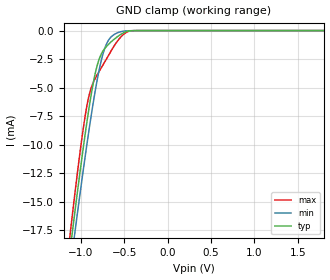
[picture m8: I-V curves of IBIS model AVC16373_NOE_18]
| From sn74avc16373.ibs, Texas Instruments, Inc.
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[Model]   AVC16373_NOE_18
Model_type  Input
Vinl=0.5775
Vinh=1.2675
| variable   typ   min   max
C_comp   1.78pF   1.31pF   2.34pF
[Temperature Range]   40   100   -40
| Ambient temperature   25   85   -40
[Voltage range]   1.8   1.65   1.95
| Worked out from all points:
|   GND clamp passes 1 mA (typ) near -0.65 V on its own axis
[GND Clamp]
| AVC16373_NOE_18
|   Voltage   I(typ)   I(min)   I(max)
-1.8V     -63.88mA   -63.41mA   -65.81mA
-1.125V   -19.32mA   -20.97mA   -17.91mA
-1.095V   -17.47mA   -19.2mA    -15.95mA
-1.065V   -15.65mA   -17.45mA   -14.03mA
-935mV    -8.251mA   -10.21mA   -6.785mA
-890mV    -6.02mA    -7.895mA   -5.239mA
-830mV    -3.604mA   -5.085mA   -4.126mA
-780mV    -2.319mA   -3.12mA    -3.454mA
-725mV    -1.575mA   -1.563mA   -2.747mA
-615mV    -751.2uA   -336.4uA   -1.327mA
-420mV    -16.5uA    -10.21uA   -21.14uA
1.8V      199.5pA    671.8pA    9.677pA
